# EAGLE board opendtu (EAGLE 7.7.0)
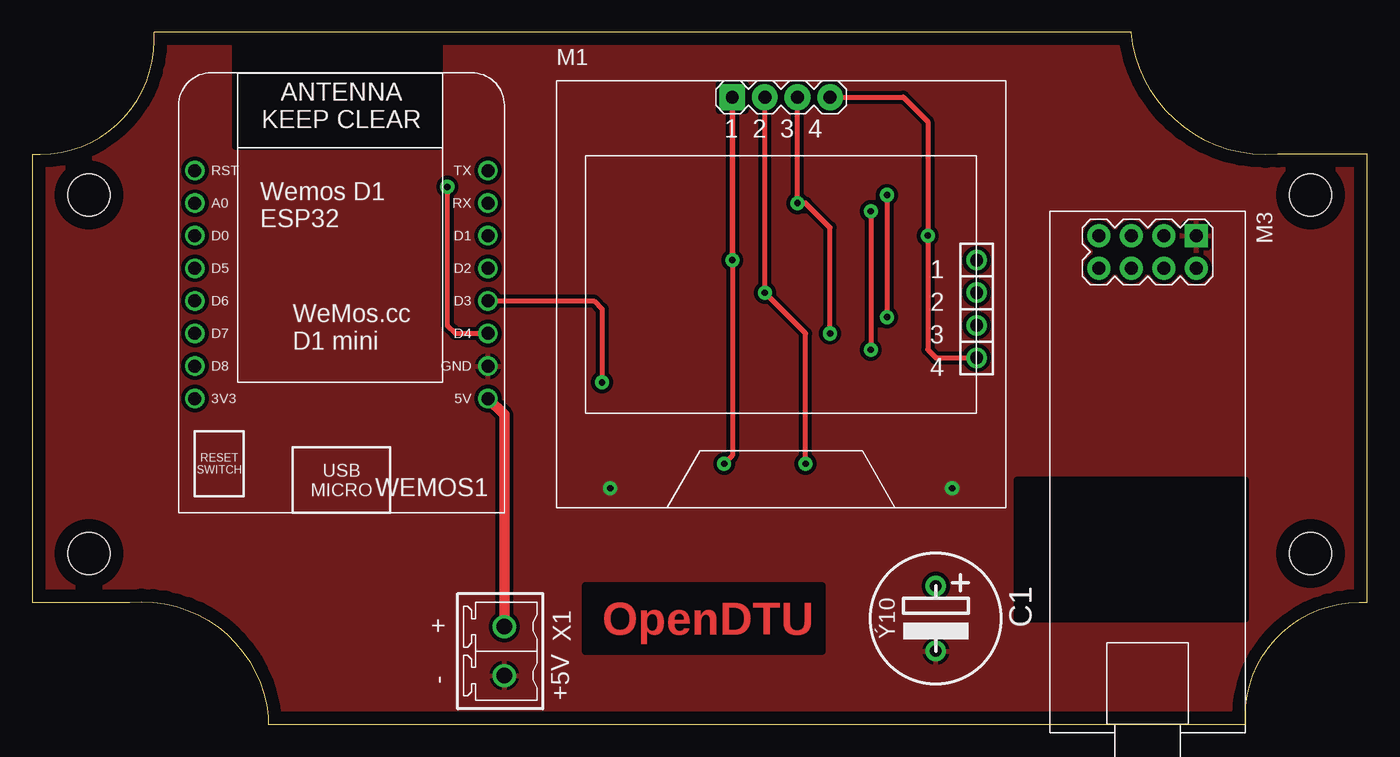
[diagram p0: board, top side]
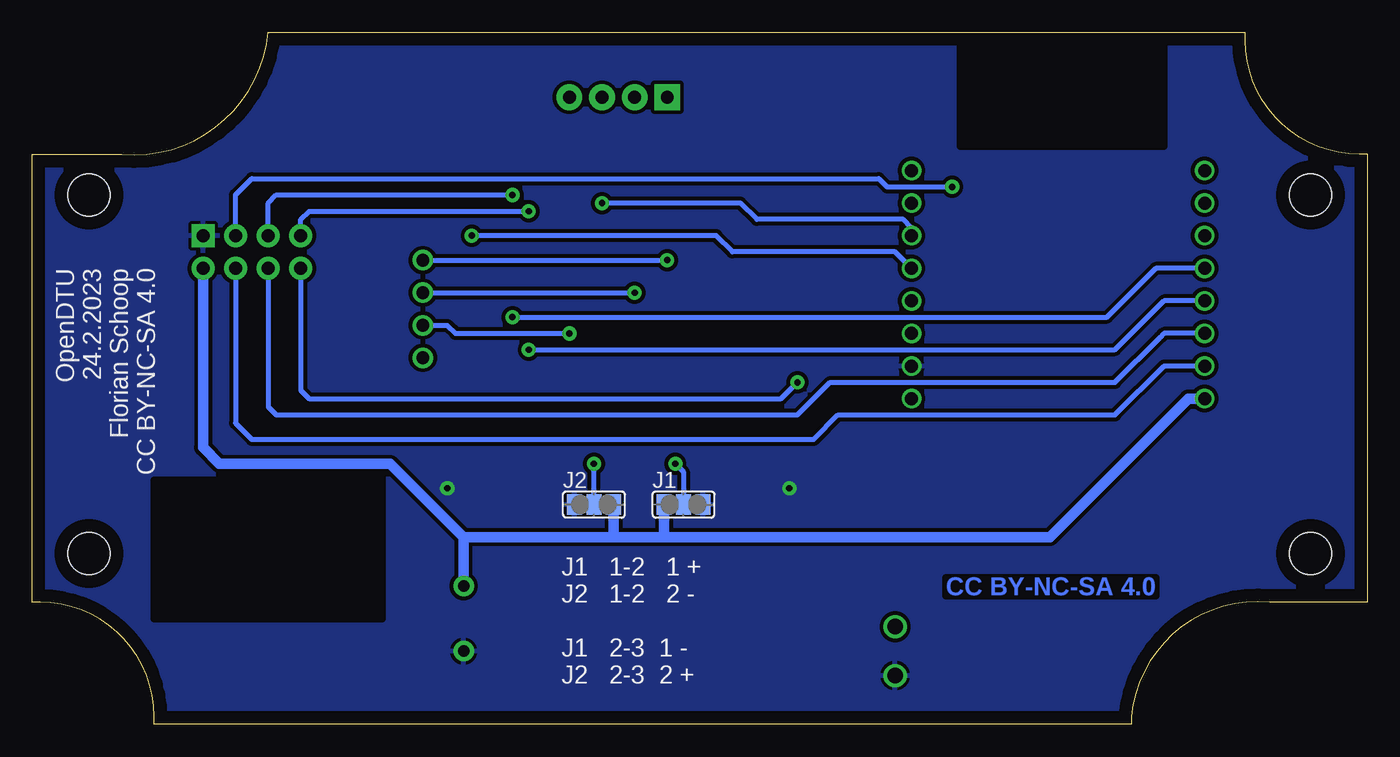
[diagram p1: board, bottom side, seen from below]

Size 104.14 x 53.98 mm. Coordinates in mm from the lower left corner, seen from the top.
Outline: 104.14,9.53 104.14,44.45 97.16,44.45 arc-90 85.72,53.98 9.53,53.98 9.53,53.34 arc-90 0.64,44.45 0,44.45 0,9.53 7.62,9.53 arc-90 18.41,0.64 18.41,0 94.61,0 94.61,0.64 arc-90 103.5,9.53 104.14,9.53
Copper layers (1*16): Component 0.035mm / dielectric 1.5mm / Solder 0.035mm
Design rules "default": minimum track width 10mil, minimum drill 0.6mm, track to track 8mil, track to pad 8mil, pad to pad 8mil, via to via 8mil, smd to smd 8mil, copper to edge 40mil, drill to drill 8mil, minimum pad ring 10mil, minimum via ring 8mil, stop-mask expansion 4mil, vias tented up to drill 0mil, thermal gap 10mil
Holes 3.3 mm at 4.45,41.27 4.45,13.34 99.69,41.27 99.69,13.34
tRestrict: area 15.9,45.1 to 31.7,54; area 76.8,8.3 to 94.6,19; area 43.2,5.7 to 61.6,10.8
bRestrict: area 15.9,45.1 to 31.7,54; area 76.8,8.3 to 94.6,19

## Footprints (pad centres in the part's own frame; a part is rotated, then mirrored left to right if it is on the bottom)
PINGERAD = drill 1 pad 1.6: 1 0,0
EB10D = drill 0.9 pad 1.6: + -2.54,0; - 2.54,0
SJ_2 = smd 1.168 x 1.6: 1 -1.524,0; 2 0,0; 3 1.524,0
DISPLAY-OLED-128X64-I2C_NH = drill 1 pad 2 square: 1 -3.81,12.7 | drill 1 pad 2: 2 -1.27,12.7; 3 1.27,12.7; 4 3.81,12.7
NRF24L01-PA-EXT = drill 1 pad 1.778 square: 1 -18.415,3.81 | drill 1.016 pad 1.778: 2 -15.875,3.81; 3 -18.415,1.27; 4 -15.875,1.27; 5 -18.415,-1.27; 6 -15.875,-1.27; 7 -18.415,-3.81; 8 -15.875,-3.81
WEMOS-D1-MINI = drill 1.016: 3V3 -10.16,-10.16; 5V 12.7,-10.16; A0 -10.16,5.08; D0 -10.16,2.54; D1 12.7,2.54; D2 12.7,0; D3 12.7,-2.54; D4 12.7,-5.08; D5 -10.16,0; D6 -10.16,-2.54; D7 -10.16,-5.08; D8 -10.16,-7.62; GND 12.7,-7.62; RESET -10.16,7.62; RX 12.7,5.08; TX 12.7,7.62
MCV1,5/2 = drill 1.2 pad 1.6: 1 0,0; 2 3.81,0

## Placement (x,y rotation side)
1  PINGERAD  [PINGERAD]  73.66,36.2 180 top
2  PINGERAD  [PINGERAD]  73.66,33.66 180 top
3  PINGERAD  [PINGERAD]  73.66,31.11 180 top
4  PINGERAD  [PINGERAD]  73.66,28.57 180 top
C1  470uF  [EB10D]  70.48,8.26 270 top
J1  [SJ_2]  53.34,17.14 0 bottom
J2  [SJ_2]  60.33,17.14 0 bottom
M1  DISPLAY-OLED-128X64-I2CNH  [DISPLAY-OLED-128X64-I2C_NH]  58.42,36.2 0 top
M3  NRF24L01-PA-EXT  [NRF24L01-PA-EXT]  86.99,19.68 270 top
WEMOS1  [WEMOS-D1-MINI]  22.86,35.56 0 top
X1  MCV1,5/2G  [MCV1,5/2]  36.83,7.62 270 top

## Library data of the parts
1-4 = 3PASSIVE
C1 = 5elko
J1 J2 = jumper_fs
M1 = EYR_Displays
M3 = EYR_Modulos
WEMOS1 = wemos d1
X1 = STECKER

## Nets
+3.3V: C1.+ J1.1 J2.3 M3.2 WEMOS1.3V3
GND: C1.- J1.3 J2.1 M3.1 WEMOS1.GND X1.2
N$1: 4.1 M1.4 WEMOS1.D2
N$2: 3.1 M1.3 WEMOS1.D1
N$3: 2.1 J2.2 M1.2
N$4: 1.1 J1.2 M1.1
N$5: M3.3 WEMOS1.D4
N$6: M3.4 WEMOS1.D8
N$7: M3.6 WEMOS1.D7
N$8: M3.7 WEMOS1.D6
N$9: M3.5 WEMOS1.D5
N$11: M3.8 WEMOS1.D3
N$12: WEMOS1.5V X1.1

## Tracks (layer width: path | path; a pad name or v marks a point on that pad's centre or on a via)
+3.3V
  Solder 0.4: 58.8,14.86 59.05,14.61 | 54.86,14.86 54.61,14.61
  Solder 0.8: 70.48,14.61 59.05,14.61 54.61,14.61 24.76,14.61 13.97,25.4 WEMOS1.3V3 | J2.3 58.8,14.86 | J1.1 54.86,14.86 | C1.+ 70.48,14.61 | M3.2 90.8,21.59 89.53,20.32 76.2,20.32 70.48,14.61
GND  (via drill 0.5 pad 1.1)
  other vias: 45.09,18.41 71.75,18.41
  pour Component (isolate 0.3): 9.53,53.98 85.72,53.98 arc90 95.25,44.45 96.52,44.45 104.14,44.45 104.14,31.75 104.14,9.53 arc90 94.61,0 73.02,0 18.41,0 arc90 8.89,9.53 5.08,9.53 0,9.53 0,12.06 0,44.45 arc90
  pour Solder (isolate 0.3): 9.53,53.98 85.72,53.98 arc90 95.25,44.45 104.14,44.45 104.14,9.53 arc90 94.61,0 59.05,0 18.41,0 arc90 8.89,9.53 0,9.53 0,26.04 0,44.45 arc90
N$1  (via drill 0.5 pad 1.1)
  Component 0.4: 4.1 70.48,28.57 69.85,29.21 v69.85,38.1 69.85,46.99 67.94,48.9 M1.4
  Solder 0.4: v69.85,38.1 50.8,38.1 49.53,36.83 36.83,36.83 WEMOS1.D2
N$2  (via drill 0.5 pad 1.1)
  Component 0.4: M1.3 v59.69,40.64 60.33,40.64 62.23,38.73 v62.23,30.48
  Solder 0.4: v59.69,40.64 48.9,40.64 47.62,39.37 36.2,39.37 35.56,38.73 WEMOS1.D1 | 3.1 71.75,31.11 71.12,30.48 v62.23,30.48
N$3  (via drill 0.5 pad 1.1)
  Component 0.4: M1.2 v57.15,33.66 60.33,30.48 v60.33,20.32
  Solder 0.4: 2.1 v57.15,33.66 | J2.2 v60.33,20.32
N$4  (via drill 0.5 pad 1.1)
  Component 0.4: v54.61,36.2 M1.1 54.61,20.95 v53.98,20.32
  Solder 0.4: 1.1 v54.61,36.2 | v53.98,20.32 53.34,19.68 J1.2
N$5  (via drill 0.5 pad 1.1)
  Component 0.4: v32.39,41.91 32.39,31.11 33.02,30.48 WEMOS1.D4
  Solder 0.4: M3.3 88.27,41.27 86.99,42.55 38.1,42.55 37.47,41.91 v32.39,41.91
N$6
  Solder 0.4: M3.4 88.27,23.49 86.99,22.22 43.18,22.22 41.27,24.13 19.68,24.13 15.88,27.94 WEMOS1.D8
N$7
  Solder 0.4: M3.6 85.72,24.76 85.09,24.13 44.45,24.13 41.91,26.67 19.68,26.67 16.19,30.16 15.88,30.48 WEMOS1.D7
N$8  (via drill 0.5 pad 1.1)
  Component 0.4: v65.41,40.01 v65.41,29.21
  Solder 0.4: M3.7 83.18,39.37 82.55,40.01 v65.41,40.01 | v65.41,29.21 19.68,29.21 15.88,33.02 WEMOS1.D6
N$9  (via drill 0.5 pad 1.1)
  Component 0.4: v66.67,41.27 v66.67,31.75
  Solder 0.4: M3.5 85.72,40.64 85.09,41.27 v66.67,41.27 | v66.67,31.75 20.32,31.75 16.51,35.56 WEMOS1.D5
N$11  (via drill 0.5 pad 1.1)
  Component 0.4: WEMOS1.D3 43.82,33.02 44.45,32.39 v44.45,26.67
  Solder 0.4: M3.8 83.18,26.04 82.55,25.4 45.72,25.4 v44.45,26.67
N$12
  Component 0.8: X1.1 36.83,24.13 WEMOS1.5V

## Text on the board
Component: OpenDTU
Solder: CC BY-NC-SA 4.0
tNames: 1 2 3 4 | Wemos D1 / ESP32 | + | - | +5V
bNames: OpenDTU / 24.2.2023 / Florian Schoop / CC BY-NC-SA 4.0 | J1 1-2 1 + / J2 1-2 2 - / / J1 2-3 1 - / J2 2-3 2 +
